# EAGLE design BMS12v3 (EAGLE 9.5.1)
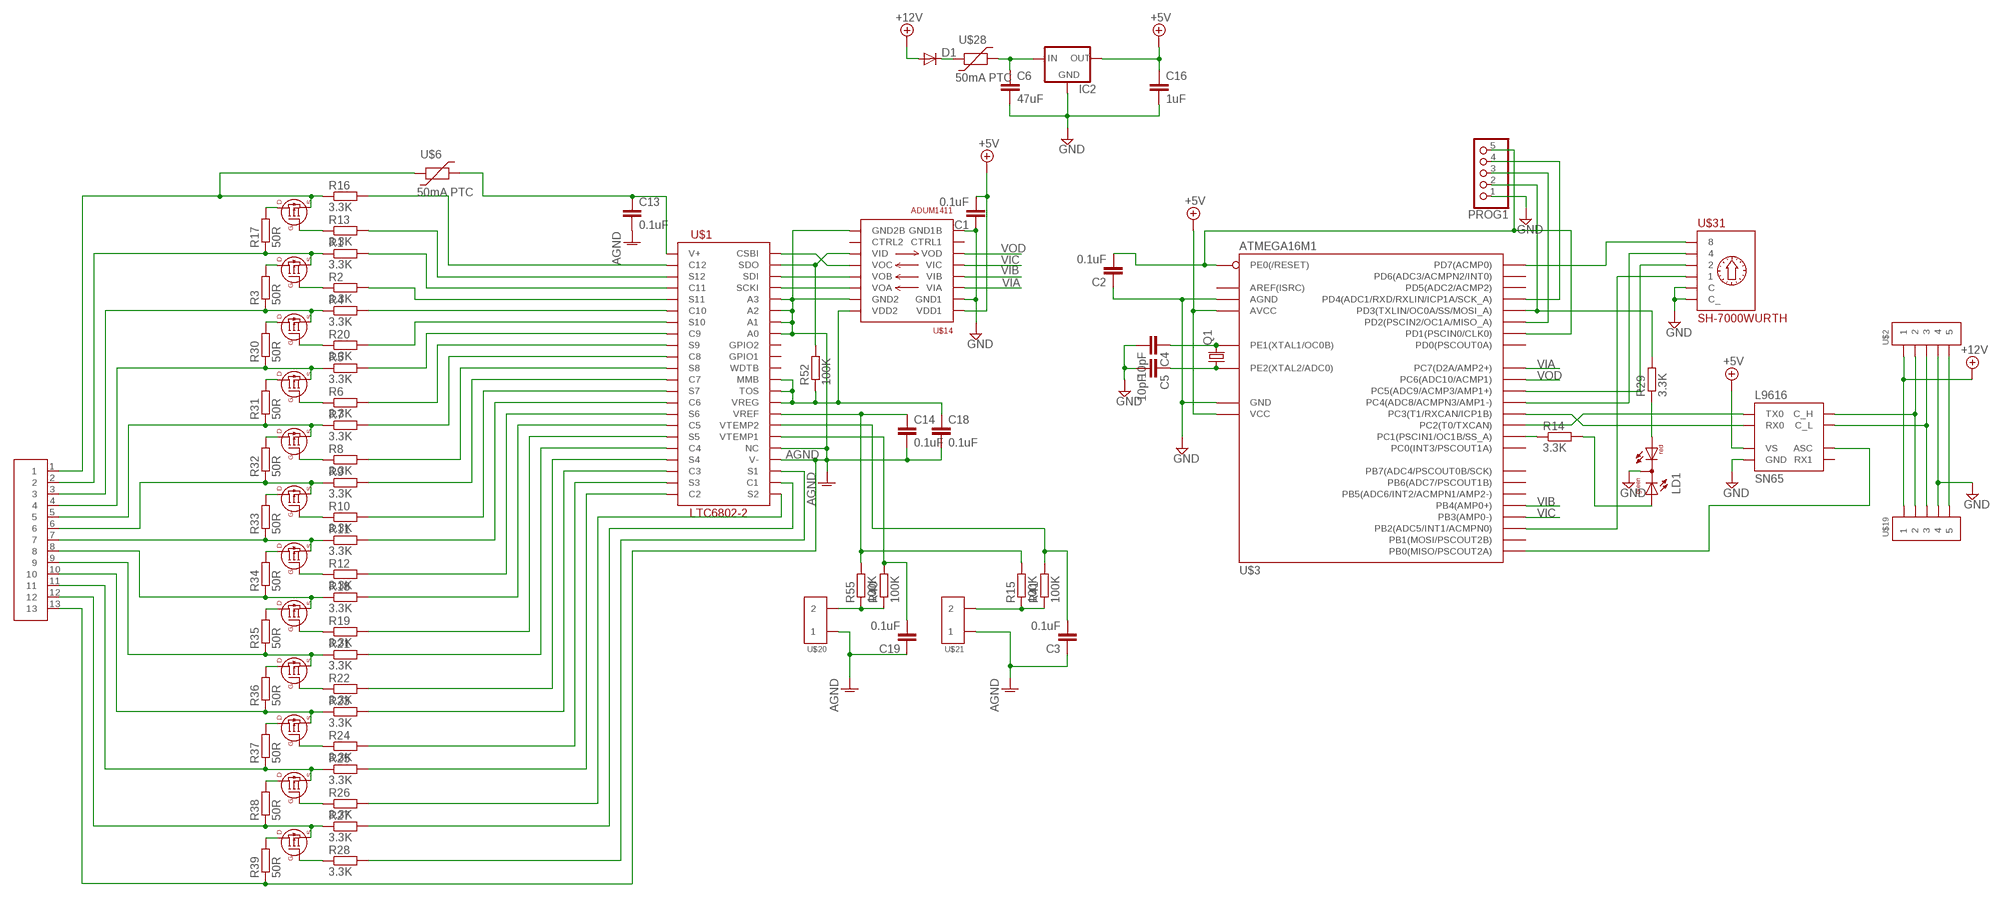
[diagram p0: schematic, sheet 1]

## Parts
C1  0.1uF  C-EUC0805  [C0805]
C2  0.1uF  C-EUC0805  [C0805]
C3  0.1uF  C-EUC0805  [C0805]
C4  10pF  C-EUC0805  [C0805]
C5  10pF  C-EUC0805  [C0805]
C6  47uF  C-EUC1206  [C1206]
C13  0.1uF  C-EUC0805  [C0805]
C14  0.1uF  C-EUC0805  [C0805]
C16  1uF  C-EUC0805  [C0805]
C18  0.1uF  C-EUC0805  [C0805]
C19  0.1uF  C-EUC0805  [C0805]
D1  DIODE-SOD123  [SOD123]
IC2  78LXXSOT89  [SOT89R]
LD1  DUOLED-RG-C  [DUOLED-C-5MM]
PROG1  PINHD-1X5  [1X05]
Q1  CRYSTALCTS406  [CTS406]
R1  3.3K  R-EU_R0805  [R0805]
R2  3.3K  R-EU_R0805  [R0805]
R3  50R  R-EU_R2512  [R2512]
R4  3.3K  R-EU_R0805  [R0805]
R5  3.3K  R-EU_R0805  [R0805]
R6  3.3K  R-EU_R0805  [R0805]
R7  3.3K  R-EU_R0805  [R0805]
R8  3.3K  R-EU_R0805  [R0805]
R9  3.3K  R-EU_R0805  [R0805]
R10  3.3K  R-EU_R0805  [R0805]
R11  3.3K  R-EU_R0805  [R0805]
R12  3.3K  R-EU_R0805  [R0805]
R13  3.3K  R-EU_R0805  [R0805]
R14  3.3K  R-EU_R0805  [R0805]
R15  100K  R-EU_R0805  [R0805]
R16  3.3K  R-EU_R0805  [R0805]
R17  50R  R-EU_R2512  [R2512]
R18  3.3K  R-EU_R0805  [R0805]
R19  3.3K  R-EU_R0805  [R0805]
R20  3.3K  R-EU_R0805  [R0805]
R21  3.3K  R-EU_R0805  [R0805]
R22  3.3K  R-EU_R0805  [R0805]
R23  3.3K  R-EU_R0805  [R0805]
R24  3.3K  R-EU_R0805  [R0805]
R25  3.3K  R-EU_R0805  [R0805]
R26  3.3K  R-EU_R0805  [R0805]
R27  3.3K  R-EU_R0805  [R0805]
R28  3.3K  R-EU_R0805  [R0805]
R29  3.3K  R-EU_R0805  [R0805]
R30  50R  R-EU_R2512  [R2512]
R31  50R  R-EU_R2512  [R2512]
R32  50R  R-EU_R2512  [R2512]
R33  50R  R-EU_R2512  [R2512]
R34  50R  R-EU_R2512  [R2512]
R35  50R  R-EU_R2512  [R2512]
R36  50R  R-EU_R2512  [R2512]
R37  50R  R-EU_R2512  [R2512]
R38  50R  R-EU_R2512  [R2512]
R39  50R  R-EU_R2512  [R2512]
R40  100K  R-EU_R0805  [R0805]
R41  100K  R-EU_R0805  [R0805]
R52  100K  R-EU_R0805  [R0805]
R55  100K  R-EU_R0805  [R0805]
SN65  L9616  [SOIC8]
U$1  LTC6802-2  [SSOP-44]
U$2  MOLEX-39502-1005  [MOLEX-39502-1005]
U$3  ATMEGA16M1  [TQFP32]
U$4  SI2351DS  [SOT23]
U$5  SI2351DS  [SOT23]
U$6  50mA PTC  1206_POLYSWITCH  [1206]
U$7  SI2351DS  [SOT23]
U$8  SI2351DS  [SOT23]
U$9  SI2351DS  [SOT23]
U$10  SI2351DS  [SOT23]
U$11  SI2351DS  [SOT23]
U$12  SI2351DS  [SOT23]
U$13  SI2351DS  [SOT23]
U$14  ADUM1411  [SOIC16W]
U$15  SI2351DS  [SOT23]
U$16  SI2351DS  [SOT23]
U$17  SI2351DS  [SOT23]
U$18  MOLEX_TERM_BLOCK_13  [MOLEX_TERM_BLOCK_13]
U$19  MOLEX-39502-1005  [MOLEX-39502-1005]
U$20  MOLEX-39502-1002  [MOLEX-39502-1002]
U$21  MOLEX-39502-1002  [MOLEX-39502-1002]
U$28  50mA PTC  1206_POLYSWITCH  [1206]
U$31  SH-7000WURTH  [WS-ROTV]

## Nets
+5V: C1.2 C16.1 IC2.2(OUT) SN65.P$3(VS) U$3.4(VCC) U$3.19(AVCC) U$14.1(VDD1)
+12V: D1.A U$2.1 U$19.1
AGND: C3.1 C13.2 C14.2 C18.2 C19.1 R39.1 U$1.26(V-) U$1.27(NC) U$1.37(A0) U$1.38(A1) U$1.39(A2) U$1.40(A3) U$14.9(GND2B) U$14.15(GND2) U$18.13 U$20.1 U$21.1
GND: C1.1 C2.1 C4.2 C5.2 C6.2 C16.2 IC2.4(GND) LD1.C PROG1.1 SN65.P$2(GND) U$2.4 U$3.5(GND) U$3.20(AGND) U$14.2(GND1) U$14.8(GND1B) U$19.4 U$31.C U$31.C2(C_)
N$1: D1.C U$28.P$1
N$2: R16.2 U$1.2(C12)
N$3: R13.2 U$1.3(S12)
N$4: R3.2 U$5.P$3(D)
N$5: R1.2 U$1.4(C11)
N$6: R1.1 R17.1 U$5.P$2(S) U$18.2
N$7: U$1.42(SDI) U$14.13(VOB)
N$8: R3.1 R4.1 U$7.P$2(S) U$18.3
N$9: R4.2 U$1.6(C10)
N$10: R26.2 U$1.23(S2)
N$11: U$1.41(SCKI) U$14.14(VOA)
N$12: R27.2 U$1.24(C1)
N$13: R28.2 U$1.25(S1)
N$14: R2.2 U$1.5(S11)
N$15: R52.2 U$1.43(SDO) U$14.11(VID)
N$16: U$1.44(CSBI) U$14.12(VOC)
N$17: R2.1 U$5.P$1(G)
N$18: R30.2 U$7.P$3(D)
N$19: C2.2 PROG1.5 U$3.31(PE0(/RESET)) U$3.32(PD1(PSCIN0/CLK0))
N$20: C6.1 IC2.1(IN) U$28.P$2
N$21: R5.2 U$1.8(C9)
N$22: R7.2 U$1.10(C8)
N$23: R9.2 U$1.12(C7)
N$24: R11.2 U$1.14(C6)
N$25: C18.1 R52.1 U$1.31(VREG) U$1.32(TOS) U$1.33(MMB) U$14.16(VDD2)
N$26: R18.2 U$1.16(C5)
N$27: R21.2 U$1.18(C4)
N$28: R23.2 U$1.20(C3)
N$29: R25.2 U$1.22(C2)
N$30: SN65.P$8(ASC) U$3.8(PB0(MISO/PSCOUT2A))
N$31: R5.1 R30.1 U$8.P$2(S) U$18.4
N$32: PROG1.2 R29.2 U$3.2(PD3(TXLIN/OC0A/SS/MOSI_A))
N$33: PROG1.3 U$3.1(PD2(PSCIN2/OC1A/MISO_A))
N$34: PROG1.4 U$3.12(PD4(ADC1/RXD/RXLIN/ICP1A/SCK_A))
N$36: SN65.P$4(RX0) U$3.7(PC3(T1/RXCAN/ICP1B))
N$37: SN65.P$1(TX0) U$3.6(PC2(T0/TXCAN))
N$38: SN65.P$7(C_H) U$2.2 U$19.2
N$39: SN65.P$6(C_L) U$2.3 U$19.3
N$40: LD1.AX(AG) R14.2
N$41: R14.1 U$3.3(PC1(PSCIN1/OC1B/SS_A))
N$42: U$3.15(PD7(ACMP0)) U$31.8
N$43: U$3.16(PB2(ADC5/INT1/ACMPN0)) U$31.1
N$44: U$3.17(PC4(ADC8/ACMPN3/AMP1-)) U$31.4
N$45: U$3.18(PC5(ADC9/ACMP3/AMP1+)) U$31.2
N$46: C3.2 R41.2 U$1.29(VTEMP2)
N$47: U$2.5 U$19.5
N$48: C4.1 Q1.3 U$3.10(PE1(XTAL1/OC0B))
N$49: C5.1 Q1.1 U$3.11(PE2(XTAL2/ADC0))
N$50: R17.2 U$4.P$3(D)
N$51: R16.1 U$4.P$2(S) U$6.P$1 U$18.1
N$52: R13.1 U$4.P$1(G)
N$53: R7.1 R31.1 U$9.P$2(S) U$18.5
N$54: R31.2 U$8.P$3(D)
N$55: R6.1 U$8.P$1(G)
N$56: R20.1 U$7.P$1(G)
N$57: R8.1 U$9.P$1(G)
N$58: R10.1 U$10.P$1(G)
N$59: R12.1 U$11.P$1(G)
N$60: R28.1 U$17.P$1(G)
N$61: R19.1 U$12.P$1(G)
N$62: R22.1 U$13.P$1(G)
N$63: R24.1 U$15.P$1(G)
N$64: R26.1 U$16.P$1(G)
N$65: R27.1 R38.1 U$17.P$2(S) U$18.12
N$66: C14.1 R15.2 R55.2 U$1.30(VREF)
N$67: C19.2 R40.2 U$1.28(VTEMP1)
N$68: LD1.AR R29.1
N$69: R25.1 R37.1 U$16.P$2(S) U$18.11
N$70: R23.1 R36.1 U$15.P$2(S) U$18.10
N$71: R38.2 U$16.P$3(D)
N$72: R39.2 U$17.P$3(D)
N$73: R37.2 U$15.P$3(D)
N$74: R21.1 R35.1 U$13.P$2(S) U$18.9
N$75: R36.2 U$13.P$3(D)
N$76: R18.1 R34.1 U$12.P$2(S) U$18.8
N$77: R35.2 U$12.P$3(D)
N$78: R11.1 R33.1 U$11.P$2(S) U$18.7
N$79: R9.1 R32.1 U$10.P$2(S) U$18.6
N$80: R33.2 U$10.P$3(D)
N$81: R34.2 U$11.P$3(D)
N$82: R32.2 U$9.P$3(D)
N$83: R24.2 U$1.21(S3)
N$84: R22.2 U$1.19(S4)
N$85: R40.1 R55.1 U$20.2
N$86: R15.1 R41.1 U$21.2
N$87: R20.2 U$1.7(S10)
N$88: R6.2 U$1.9(S9)
N$89: R8.2 U$1.11(S8)
N$90: R10.2 U$1.13(S7)
N$91: R12.2 U$1.15(S6)
N$93: R19.2 U$1.17(S5)
V+: C13.1 U$1.1(V+) U$6.P$2
VIA: U$3.25(PC7(D2A/AMP2+)) U$14.3(VIA)
VIB: U$3.24(PB4(AMP0+)) U$14.4(VIB)
VIC: U$3.23(PB3(AMP0-)) U$14.5(VIC)
VOD: U$3.22(PC6(ADC10/ACMP1)) U$14.6(VOD)
Unconnected: SN65.P$5(RX1) U$1.34(WDTB) U$1.35(GPIO1) U$1.36(GPIO2) U$3.9(PB1(MOSI/PSCOUT2B)) U$3.13(PD5(ADC2/ACMP2)) U$3.14(PD6(ADC3/ACMPN2/INT0)) U$3.21(AREF(ISRC)) U$3.26(PB5(ADC6/INT2/ACMPN1/AMP2-)) U$3.27(PB6(ADC7/PSCOUT1B)) U$3.28(PB7(ADC4/PSCOUT0B/SCK)) U$3.29(PD0(PSCOUT0A)) U$3.30(PC0(INT3/PSCOUT1A)) U$14.7(CTRL1) U$14.10(CTRL2)

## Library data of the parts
C1-C6 C13 C14 C16 C18 C19 = resistor:C-EU: CAPACITOR, European symbol
D1 = diode:DIODE-: DIODE
IC2 = v-reg:78LXX: VOLTAGE REGULATOR
LD1 = led:DUOLED-RG-C: DUO LED 2 colors (red/green), 5 mm, round, common Cathode www.ligitek.com or other producers.
PROG1 = pinhead:PINHD-1X5: PIN HEADER
Q1 = crystal:CRYSTAL: CRYSTAL
R1-R41 R52 R55 = resistor:R-EU_: RESISTOR, European symbol
SN65 = Ians parts:L9616
U$1 = Ians parts:LTC6802-2
U$2 U$19 = Ians parts:MOLEX-39502-1005
U$3 = Ians parts:ATMEGA16M1
U$4 U$5 U$7-U$13 U$15-U$17 = Ians parts:SI2351DS
U$6 U$28 = Ians parts:1206_POLYSWITCH
U$14 = Ians parts:ADUM1411
U$18 = Ians parts:MOLEX_TERM_BLOCK_13
U$20 U$21 = Ians parts:MOLEX-39502-1002
U$31 = Ians parts:SH-7000

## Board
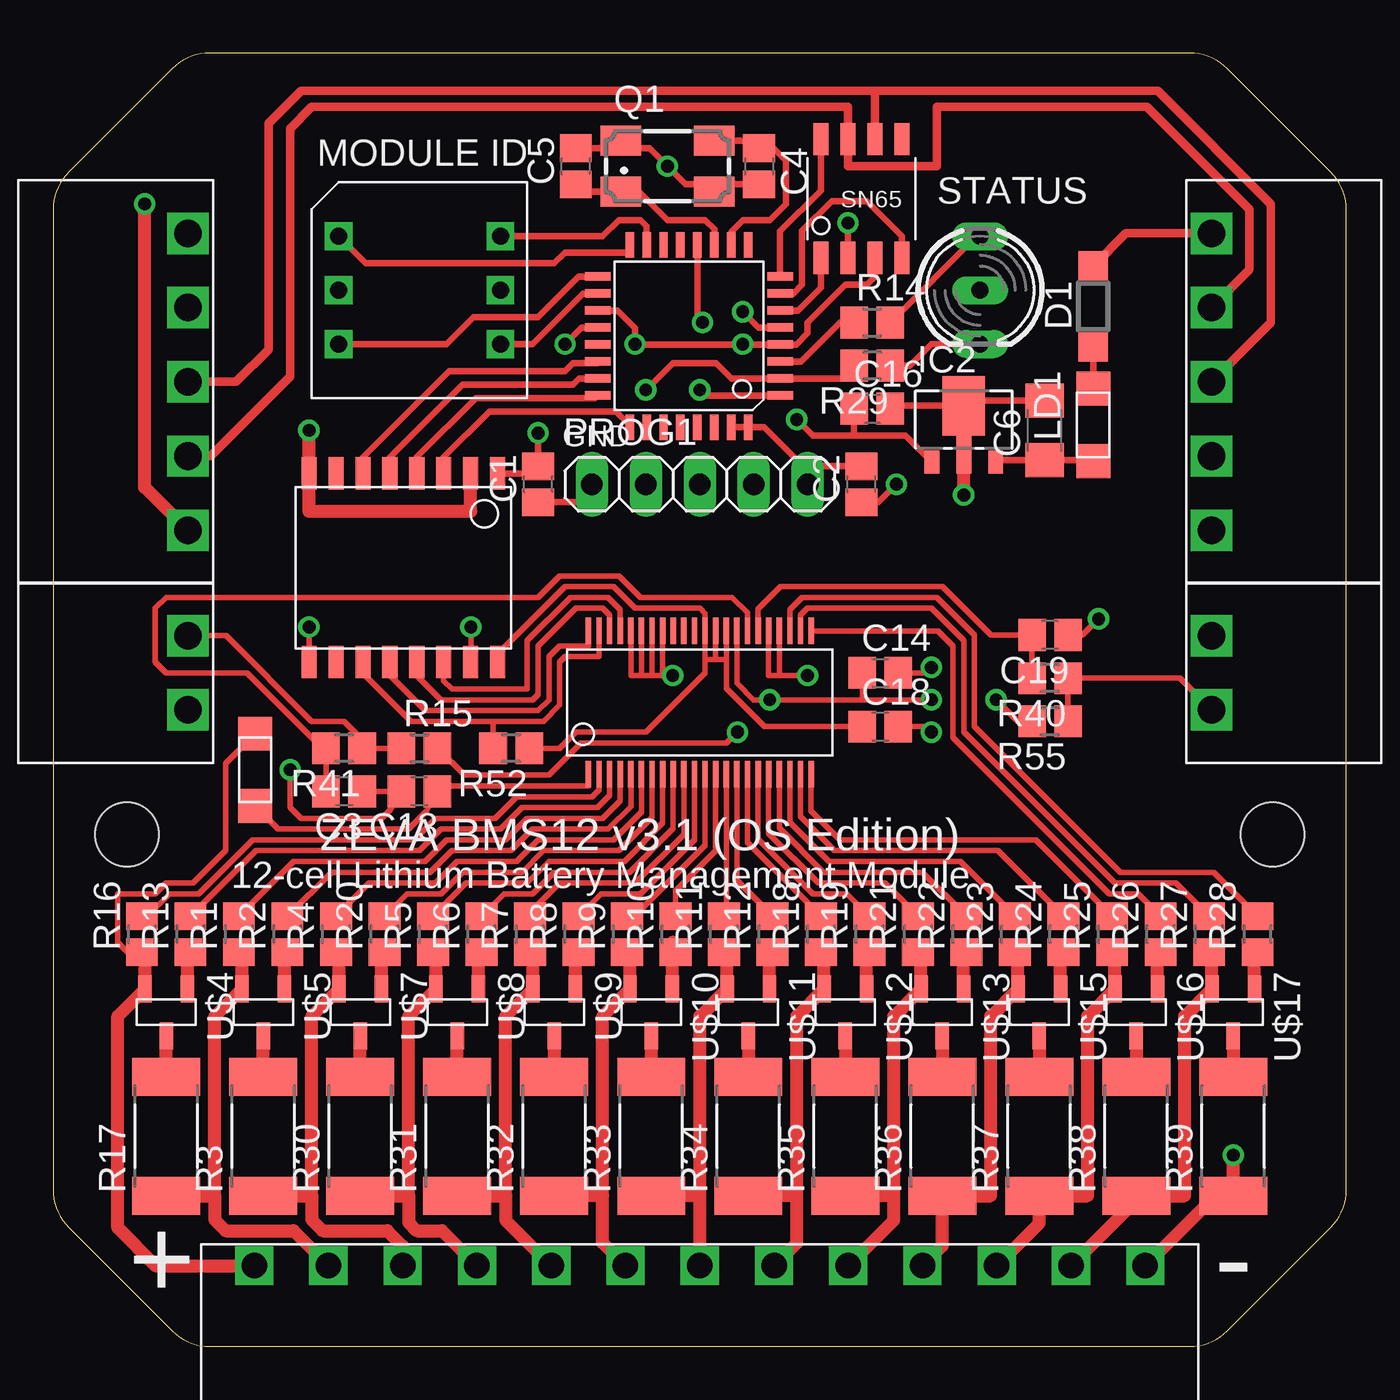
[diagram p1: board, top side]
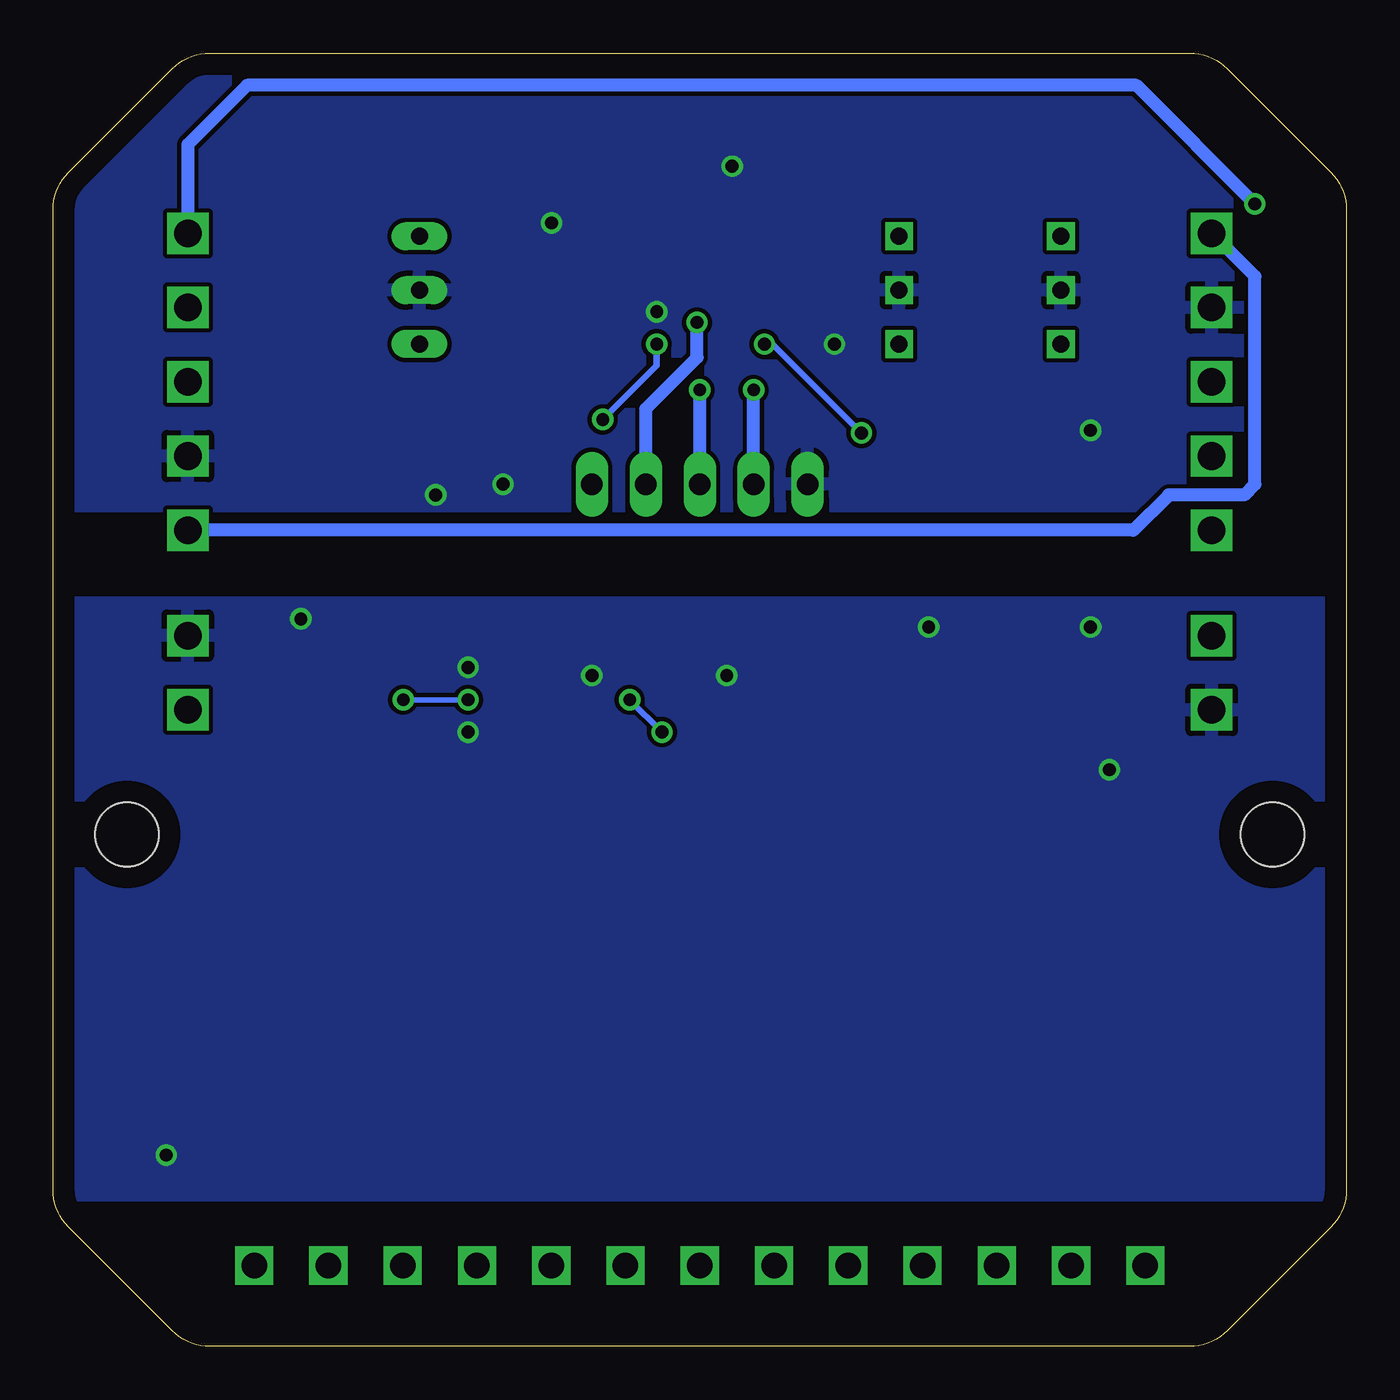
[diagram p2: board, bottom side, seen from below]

Size 60.96 x 60.96 mm. Coordinates in mm from the lower left corner, seen from the top.
Outline: 5.61,0.74 arc45 7.4,0 53.56,0 arc45 55.35,0.74 60.22,5.61 arc45 60.96,7.4 60.96,53.56 arc45 60.22,55.35 55.35,60.22 arc45 53.56,60.96 7.4,60.96 arc45 5.61,60.22 0.74,55.35 arc45 0,53.56 0,7.4 arc45 0.74,5.61 5.61,0.74
Copper layers (1*16): Top 0.035mm / dielectric 1.5mm / Bottom 0.035mm
Design rules "default *": minimum track width 10mil, minimum drill 10mil, track to track 8mil, track to pad 8mil, pad to pad 8mil, via to via 8mil, smd to smd 8mil, copper to edge 40mil, drill to drill 8mil, minimum pad ring 10mil, minimum via ring 8mil, stop-mask expansion 4mil, vias tented up to drill 0mil, thermal gap 10mil
Holes 3 mm at 3.48,24.13 57.48,24.13

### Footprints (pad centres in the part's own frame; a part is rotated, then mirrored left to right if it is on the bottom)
C0805 = smd 1.3 x 1.5: 1 -0.85,0; 2 0.85,0
C1206 = smd 1.6 x 1.8: 1 -1.4,0; 2 1.4,0
SOD123 = smd 1.4 x 1.4: A 1.9,0; C -1.9,0
SOT89R = smd 0.7 x 1.1: 1 1.5,-1.75; 2 -1.5,-1.75 | smd 0.7 x 1.8: 3 0,-1.4 | smd 2 x 2.8: 4 0,0.9
DUOLED-C-5MM = drill 0.813 long: AR 2.54,0; AX -2.54,0; C 0,0
1X05 = drill 1.016 long: 1 -5.08,0; 2 -2.54,0; 3 0,0; 4 2.54,0; 5 5.08,0
CTS406 = smd 1.9 x 1.4: 1 -2.2,-1.2; 2 2.2,-1.2; 3 2.2,1.2; 4 -2.2,1.2
R0805 = smd 1.3 x 1.5: 1 -0.85,0; 2 0.85,0
R2512 = smd 1.8 x 3.2: 1 -2.8,0; 2 2.8,0
SOIC8 = smd 1.524 x 0.711: P$1 -2.794,1.905; P$2 -2.794,0.635; P$3 -2.794,-0.635; P$4 -2.794,-1.905; P$5 2.794,-1.905; P$6 2.794,-0.635; P$7 2.794,0.635; P$8 2.794,1.905
SSOP-44 = smd 1.25 x 0.25: 1 -3.375,5.25; 2 -3.375,4.75; 3 -3.375,4.25; 4 -3.375,3.75; 5 -3.375,3.25; 6 -3.375,2.75; 7 -3.375,2.25; 8 -3.375,1.75; 9 -3.375,1.25; 10 -3.375,0.75; 11 -3.375,0.25; 12 -3.375,-0.25; 13 -3.375,-0.75; 14 -3.375,-1.25; 15 -3.375,-1.75; 16 -3.375,-2.25; 17 -3.375,-2.75; 18 -3.375,-3.25; 19 -3.375,-3.75; 20 -3.375,-4.25; 21 -3.375,-4.75; 22 -3.375,-5.25; 23 3.375,-5.25; 24 3.375,-4.75; 25 3.375,-4.25; 26 3.375,-3.75; 27 3.375,-3.25; 28 3.375,-2.75; 29 3.375,-2.25; 30 3.375,-1.75; 31 3.375,-1.25; 32 3.375,-0.75; 33 3.375,-0.25; 34 3.375,0.25; 35 3.375,0.75; 36 3.375,1.25; 37 3.375,1.75; 38 3.375,2.25; 39 3.375,2.75; 40 3.375,3.25; 41 3.375,3.75; 42 3.375,4.25; 43 3.375,4.75; 44 3.375,5.25
MOLEX-39502-1005 = drill 1.3 square: 1 -7,0; 2 -3.5,0; 3 0,0; 4 3.5,0; 5 7,0
TQFP32 = smd 1.2 x 0.4: 1 -4.3,2.8; 2 -4.3,2; 3 -4.3,1.2; 4 -4.3,0.4; 5 -4.3,-0.4; 6 -4.3,-1.2; 7 -4.3,-2; 8 -4.3,-2.8; 17 4.3,-2.8; 18 4.3,-2; 19 4.3,-1.2; 20 4.3,-0.4; 21 4.3,0.4; 22 4.3,1.2; 23 4.3,2; 24 4.3,2.8 | smd 0.4 x 1.2: 9 -2.8,-4.3; 10 -2,-4.3; 11 -1.2,-4.3; 12 -0.4,-4.3; 13 0.4,-4.3; 14 1.2,-4.3; 15 2,-4.3; 16 2.8,-4.3; 25 2.8,4.3; 26 2,4.3; 27 1.2,4.3; 28 0.4,4.3; 29 -0.4,4.3; 30 -1.2,4.3; 31 -2,4.3; 32 -2.8,4.3
SOT23 = smd 1.27 x 0.635: P$1 -1.1,1; P$2 -1.1,-1; P$3 1.1,0
1206 = smd 1.6 x 1.6: P$1 -1.7,0; P$2 1.7,0
SOIC16W = smd 1.524 x 0.711: 1 -4.445,4.445; 2 -4.445,3.175; 3 -4.445,1.905; 4 -4.445,0.635; 5 -4.445,-0.635; 6 -4.445,-1.905; 7 -4.445,-3.175; 8 -4.445,-4.445; 9 4.445,-4.445; 10 4.445,-3.175; 11 4.445,-1.905; 12 4.445,-0.635; 13 4.445,0.635; 14 4.445,1.905; 15 4.445,3.175; 16 4.445,4.445
MOLEX_TERM_BLOCK_13 = drill 1.2 square: 1 -21,0; 2 -17.5,0; 3 -14,0; 4 -10.5,0; 5 -7,0; 6 -3.5,0; 7 0,0; 8 3.5,0; 9 7,0; 10 10.5,0; 11 14,0; 12 17.5,0; 13 21,0
MOLEX-39502-1002 = drill 1.3 square: 1 -1.75,0; 2 1.75,0
WS-ROTV = drill 0.8 square: 1 -3.81,2.54; 2 3.81,-2.54; 4 -3.81,-2.54; 8 3.81,2.54; C -3.81,0; C2 3.81,0

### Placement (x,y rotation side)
C1  22.86,40.64 90 top
C2  38.1,40.64 90 top
C3  13.72,26.16 180 top
C4  33.27,55.63 270 top
C5  24.64,55.63 90 top
C6  46.74,43.18 90 top
C13  17.27,26.16 180 top
C14  38.99,31.75 0 top
C16  38.61,44.2 0 top
C18  38.99,29.21 0 top
C19  46.99,33.53 180 top
D1  49.02,49.02 90 top
IC2  42.93,43.43 0 top
LD1  43.69,49.78 270 top
PROG1  30.48,40.64 0 top
Q1  28.96,55.63 0 top
R1  8.76,19.43 90 top
R2  11.05,19.43 90 top
R3  9.91,9.91 90 top
R4  13.34,19.43 90 top
R5  17.91,19.43 90 top
R6  20.19,19.43 90 top
R7  22.48,19.43 90 top
R8  24.77,19.43 90 top
R9  27.05,19.43 90 top
R10  29.34,19.43 90 top
R11  31.62,19.43 90 top
R12  33.91,19.43 90 top
R13  6.48,19.43 90 top
R14  38.61,48.26 0 top
R15  17.27,28.19 0 top
R16  4.19,19.43 90 top
R17  5.33,9.91 90 top
R18  36.2,19.43 90 top
R19  38.48,19.43 90 top
R20  15.62,19.43 90 top
R21  40.77,19.43 90 top
R22  43.05,19.43 90 top
R23  45.34,19.43 90 top
R24  47.62,19.43 90 top
R25  49.91,19.43 90 top
R26  52.2,19.43 90 top
R27  54.48,19.43 90 top
R28  56.77,19.43 90 top
R29  38.61,46.23 180 top
R30  14.48,9.91 90 top
R31  19.05,9.91 90 top
R32  23.62,9.91 90 top
R33  28.19,9.91 90 top
R34  32.77,9.91 90 top
R35  37.34,9.91 90 top
R36  41.91,9.91 90 top
R37  46.48,9.91 90 top
R38  51.05,9.91 90 top
R39  55.63,9.91 90 top
R40  46.99,31.5 180 top
R41  13.72,28.19 180 top
R52  21.59,28.19 180 top
R55  46.99,29.46 180 top
SN65  38.1,54.1 90 top
U$1  30.48,30.35 90 top
U$2  6.35,45.47 90 top
U$3  29.97,47.62 180 top
U$4  5.33,15.75 270 top
U$5  9.91,15.75 270 top
U$6  9.53,27.18 270 top
U$7  14.48,15.75 270 top
U$8  19.05,15.75 270 top
U$9  23.62,15.75 270 top
U$10  28.19,15.75 270 top
U$11  32.77,15.75 270 top
U$12  37.34,15.75 270 top
U$13  41.91,15.75 270 top
U$14  16.51,36.7 270 top
U$15  46.48,15.75 270 top
U$16  51.05,15.75 270 top
U$17  55.63,15.75 270 top
U$18  30.48,3.81 0 top
U$19  54.61,45.47 270 top
U$20  54.61,31.75 270 top
U$21  6.35,31.75 90 top
U$28  49.02,43.43 270 top
U$31  17.27,49.78 0 top

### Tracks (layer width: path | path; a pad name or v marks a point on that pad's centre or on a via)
+5V  (via drill 0.6)
  Top 0.305: v22.86,43.05 C1.2 22.86,41.15 U$14.1 | SN65.P$3 38.73,50.42 38.35,50.04 37.34,50.04 35.56,48.26 35.56,47.75 35.03,47.23 U$3.4 32.51,47.23 | U$3.19 26.61,48.83 27.43,48.01 v27.43,47.24 27.45,47.23 32.51,47.23 | 32.51,47.23 v32.51,47.24 | v35.05,43.69 35.81,42.93 36.58,42.93 37.76,42.93 | 37.76,42.93 40.18,42.93 IC2.2 | 37.76,42.93 C16.1
  Bottom 0.305: v27.43,47.24 27.05,47.24 v22.86,43.05 | v32.51,47.24 32.51,46.23 v35.05,43.69
+12V  (via drill 0.6)
  Top 0.406: U$19.1 50.57,52.47 D1.A
  Top 0.61: U$2.1 4.32,40.5 v4.32,53.85
  Bottom 0.61: v4.32,53.85 9.91,59.44 51.82,59.44 54.61,56.64 U$19.1
AGND  (via drill 0.6)
  Top 0.254: 34.23,31.62 U$1.26 | 34.23,31.62 v35.56,31.62 | U$1.27 33.73,31.62 34.23,31.62 | U$1.37 28.73,31.62 v29.21,31.62 | U$1.38 28.23,31.62 v29.21,31.62 | U$1.39 27.73,31.62 v29.21,31.62 | U$1.40 27.23,31.62 v29.21,31.62 | U$14.15 v19.69,33.91 | U$14.9 v12.06,33.91 | C14.2 41.15,31.75 v41.4,32 | C18.2 41.15,29.21 v41.4,28.96 | C19.1 48.51,33.53 v49.28,34.29 | C3.1 C13.2 15.91,25.31 15.49,24.89 11.68,24.89 11.18,25.4 v11.18,27.18
  Top 0.61: U$18.13 54.78,7.11 R39.1 v55.63,9.02
  Bottom 0.61: v12.06,33.91 11.81,33.91
  pour Bottom: -1.52,7.11 61.98,7.11 62.23,35.05 -1.27,35.05
GND  (via drill 0.6)
  Top 0.305: U$3.5 33.26,48.02 v32.51,48.77 | SN65.P$2 v37.47,52.96 | v39.75,40.64 38.9,39.79 C2.1 | C1.1 25.4,39.79 PROG1.1 | C5.2 28.11,56.48 v28.96,55.63 29.81,54.78 C4.2 | C6.2 43.17,44.58 IC2.4 39.46,44.33 C16.2 | U$3.20 24.91,48.02 v24.13,47.24
  Top 0.61: U$14.2 19.68,39.37 12.06,39.37 U$14.8 v12.06,43.18 | v42.93,40.13 IC2.4
  pour Bottom: -1.27,39.62 -1.27,62.23 62.23,62.23 62.23,39.62
N$1
  Top 0.305: U$28.P$1 D1.C
N$2
  Top 0.254: U$1.2 25.73,26.24 25.4,25.91 21.84,25.91 20.83,24.89 18.03,24.89 17.02,23.88 9.4,23.88 6.86,21.34 5.5,21.34 4.45,20.28 R16.2
N$3
  Top 0.254: U$1.3 26.23,25.98 25.65,25.4 22.1,25.4 21.08,24.38 18.29,24.38 17.27,23.37 9.56,23.37 R13.2
N$4
  Top 0.61: R3.2 U$5.P$3
N$5
  Top 0.254: U$1.4 26.73,25.71 25.91,24.89 22.35,24.89 21.34,23.88 18.54,23.88 17.53,22.86 11.34,22.86 R1.2
N$6
  Top 0.61: U$18.2 11.33,5.46 8.13,5.46 7.62,5.97 7.62,7.11 | 7.62,7.11 7.62,15.56 U$5.P$2 8.91,18.44 R1.1 | R17.1 7.62,7.11
N$7
  Top 0.254: U$1.42 26.23,34.48 25.91,34.8 24.64,34.8 22.86,33.02 22.86,30.73 22.61,30.48 18.29,30.48 17.14,31.62 U$14.13
N$8
  Top 0.61: 12.19,7.11 12.19,15.56 U$7.P$2 13.48,18.44 R4.1 | U$18.3 16.48,4.73 15.75,5.46 12.7,5.46 12.19,5.97 12.19,7.11 | R3.1 12.19,7.11
N$9
  Top 0.254: U$1.6 27.73,25.19 26.42,23.88 22.86,23.88 21.84,22.86 19.05,22.86 18.03,21.84 14.9,21.84 R4.2
N$10
  Top 0.254: U$1.23 41.71,33.73 42.42,33.02 42.42,28.7 49.78,21.34 51.14,21.34 R26.2
N$11
  Top 0.254: U$1.41 26.73,34.74 26.16,35.31 24.38,35.31 22.35,33.27 22.35,30.99 18.8,30.99 18.41,31.37 U$14.14
N$12
  Top 0.254: U$1.24 35.23,34.47 35.56,34.8 41.4,34.8 42.93,33.27 42.93,28.96 50.04,21.84 52.92,21.84 R27.2
N$13
  Top 0.254: U$1.25 34.73,34.73 35.31,35.31 41.66,35.31 43.43,33.53 43.43,29.21 50.29,22.35 54.7,22.35 R28.2
N$14
  Top 0.254: U$1.5 27.23,25.45 26.16,24.38 22.61,24.38 21.59,23.37 18.8,23.37 17.78,22.35 13.12,22.35 R2.2
N$15
  Top 0.254: U$1.43 25.73,32.51 24.13,32.51 23.88,32.26 23.88,30.23 23.11,29.46 20.74,29.46 | U$14.11 14.61,31.73 16.87,29.46 20.74,29.46 | 20.74,29.46 R52.2
N$16
  Top 0.254: U$1.44 25.23,33.02 23.88,33.02 23.37,32.51 23.37,30.48 22.86,29.97 17.53,29.97 15.88,31.62 U$14.12
N$17
  Top 0.61: R2.1 10.91,18.44 U$5.P$1
N$18
  Top 0.61: R30.2 U$7.P$3
N$19
  Top 0.305: U$3.31 U$3.32 33.51,43.33 35.56,41.27 PROG1.5 35.56,41.49 C2.2
N$20
  Top 0.305: U$28.P$2 48.98,41.78 C6.1 44.52,41.78 IC2.1
N$21
  Top 0.254: U$1.8 28.73,24.67 26.92,22.86 23.37,22.86 22.35,21.84 19.47,21.84 R5.2
N$22
  Top 0.254: U$1.10 29.73,24.14 27.43,21.84 23.88,21.84 22.48,20.45 R7.2
N$23
  Top 0.254: U$1.12 30.73,23.62 27.69,20.57 27.34,20.57 R9.2
N$24
  Top 0.254: U$1.14 31.73,20.39 R11.2
N$25
  Top 0.254: 31.73,32.38 U$1.31 | 31.23,32.38 U$1.32 | 31.23,32.38 31.73,32.38 | 30.73,32.38 U$1.33 30.73,34.55 30.48,34.8 27.43,34.8 26.42,35.81 24.13,35.81 20.95,32.64 U$14.16 | 30.73,32.38 31.23,32.38 | 30.73,32.38 30.73,31.75 27.94,28.96 24.64,28.96 23.88,28.19 R52.1 | C18.1 33.53,29.21 31.73,31.01 31.73,32.38
N$26
  Top 0.254: U$1.16 32.73,23.75 R18.2
N$27
  Top 0.254: U$1.18 33.73,24.18 36.07,21.84 39.2,21.84 R21.2
N$28
  Top 0.254: U$1.20 34.73,24.71 36.58,22.86 42.76,22.86 R23.2
N$29
  Top 0.254: U$1.22 35.73,25.23 37.08,23.88 46.32,23.88 R25.2
N$30
  Top 0.305: SN65.P$8 36.2,54.48 34.27,52.56 U$3.8
N$31
  Top 0.61: 16.76,7.11 16.76,15.56 U$8.P$2 18.05,18.44 R5.1 | U$18.4 18.33,5.46 17.14,5.46 16.76,5.84 16.76,7.11 | R30.1 16.76,7.11
N$32  (via drill 0.6)
  Top 0.305: v27.94,45.09 29.21,46.35 31.24,46.35 31.97,45.62 U$3.2 37.16,45.62 R29.2
  Bottom 0.61: PROG1.2 v27.94,45.09
N$33  (via drill 0.6)
  Top 0.305: U$3.1 30.73,44.83 v30.48,45.09
  Bottom 0.61: PROG1.3 v30.48,45.09
N$34  (via drill 0.6)
  Top 0.305: U$3.12 30.37,48.49 v30.61,48.26
  Bottom 0.61: PROG1.4 33.02,44.2 30.61,46.61 v30.61,48.26
N$36
  Top 0.305: SN65.P$4 40.01,52.32 38.35,53.98 36.7,53.98 35.31,52.58 35.31,50.04 34.89,49.62 U$3.7
N$37
  Top 0.305: U$3.6 35.11,48.83 36.2,49.91 SN65.P$1
N$38
  Top 0.406: U$2.2 7.42,41.97 11.18,45.72 11.18,57.4 12.19,58.42 37.47,58.42 SN65.P$7 37.47,55.63 41.66,55.63 41.66,58.42 51.56,58.42 56.39,53.59 56.39,50.74 U$19.2
N$39
  Top 0.406: 38.73,59.18 SN65.P$6 | 38.73,59.18 52.07,59.18 57.4,53.85 57.4,48.26 U$19.3 | U$2.3 8.64,45.47 10.16,46.99 10.16,57.66 11.68,59.18 38.73,59.18
N$40
  Top 0.305: LD1.AX 43.52,52.32 R14.2
N$41
  Top 0.305: R14.1 37.08,48.26 35.25,46.42 U$3.3
N$42
  Top 0.305: U$3.15 27.97,52.8 27.69,53.09 26.67,53.09 25.91,52.32 U$31.8
N$43
  Top 0.305: U$31.1 14.73,51.05 23.62,51.05 24.13,51.56 27.17,51.56 U$3.16
N$44
  Top 0.305: U$3.17 24.77,50.42 22.86,48.51 19.81,48.51 18.54,47.24 U$31.4
N$45
  Top 0.305: U$3.18 24.99,49.62 22.61,47.24 U$31.2
N$46
  Top 0.254: U$1.29 32.73,34.58 32,35.31 27.69,35.31 26.67,36.32 23.88,36.32 22.86,35.31 5.33,35.31 4.83,34.8 4.83,32.26 5.33,31.75 9.14,31.75 12.7,28.19 R41.2 | R41.2 C3.2 | R41.2 12.7,27.69
N$47
  Bottom 0.61: U$19.5 10.05,38.47 8.38,40.13 4.83,40.13 4.32,40.64 4.32,50.43 U$2.5
N$48
  Top 0.305: Q1.3 33.05,56.83 C4.1 33.95,56.48 34.54,55.88 34.54,53.85 33.78,53.09 32.51,53.09 31.97,52.55 U$3.10
N$49
  Top 0.305: U$3.11 31.17,52.65 30.73,53.09 28.96,53.09 27.62,54.43 Q1.1 24.99,54.43 C5.1
N$50
  Top 0.61: R17.2 U$4.P$3
N$51
  Top 0.254: R16.1 3.52,18.58 3.05,19.05 3.05,21.34 4.83,21.34 5.33,21.84 6.6,21.84 8.13,23.37 8.13,27.48 U$6.P$1
  Top 0.61: U$18.1 4.83,3.81 3.05,5.59 3.05,15.56 U$4.P$2 4.33,18.44 R16.1
N$52
  Top 0.61: R13.1 6.33,18.44 U$4.P$1
N$53
  Top 0.61: 21.34,7.11 21.34,15.56 U$9.P$2 22.62,18.44 R7.1 | U$18.5 21.34,5.95 21.34,7.11 | R31.1 21.34,7.11
N$54
  Top 0.61: R31.2 U$8.P$3
N$55
  Top 0.61: R6.1 20.05,18.44 U$8.P$1
N$56
  Top 0.61: R20.1 15.48,18.44 U$7.P$1
N$57
  Top 0.61: R8.1 24.62,18.44 U$9.P$1
N$58
  Top 0.61: R10.1 29.21,18.71 29.21,19.05 29.19,19.03 U$10.P$1
N$59
  Top 0.61: R12.1 33.77,18.44 U$11.P$1
N$60
  Top 0.61: R28.1 56.63,18.44 U$17.P$1
N$61
  Top 0.61: R19.1 38.34,18.44 U$12.P$1
N$62
  Top 0.61: R22.1 42.91,18.44 U$13.P$1
N$63
  Top 0.61: R24.1 47.48,18.44 U$15.P$1
N$64
  Top 0.61: R26.1 52.05,18.44 U$16.P$1
N$65
  Top 0.61: U$18.12 51.05,6.88 R38.1 53.34,7.11 53.34,15.56 U$17.P$2 54.63,18.44 R27.1
N$66  (via drill 0.6)
  Top 0.254: U$1.30 32.23,31.27 33.02,30.48 v33.78,30.48 38.14,30.48 | 38.14,30.48 v41.4,30.48 | 38.14,30.48 C14.1 | R55.2 45.47,29.46 v44.45,30.48 | v32.26,28.96 31.75,28.45 24.89,28.45 23.37,26.92 19.39,26.92 R15.2
  Bottom 0.254: v41.4,30.48 v44.45,30.48 | v32.26,28.96 v33.78,30.48
N$67
  Top 0.254: U$1.28 33.23,34.75 34.29,35.81 41.91,35.81 44.2,33.53 C19.2 R40.2
N$68
  Top 0.305: LD1.AR 41.4,47.24 40.39,46.23 R29.1
N$69
  Top 0.61: U$18.11 46.48,5.81 R37.1 48.77,7.11 48.77,15.56 U$16.P$2 50.05,18.44 R25.1
N$70
  Top 0.61: U$18.10 41.91,4.74 R36.1 44.2,7.11 44.2,15.56 U$15.P$2 45.48,18.44 R23.1
N$71
  Top 0.61: U$16.P$3 R38.2
N$72
  Top 0.61: U$17.P$3 R39.2
N$73
  Top 0.61: U$15.P$3 R37.2
N$74
  Top 0.61: 39.62,7.11 39.62,5.95 U$18.9 | 39.62,7.11 R35.1 | 39.62,7.11 39.62,15.56 U$13.P$2 40.91,18.44 R21.1
N$75
  Top 0.61: U$13.P$3 R36.2
N$76
  Top 0.61: 35.05,7.11 35.05,15.56 U$12.P$2 36.34,18.44 R18.1 | U$18.8 35.05,4.88 35.05,7.11 | 35.05,7.11 R34.1
N$77
  Top 0.61: U$12.P$3 R35.2
N$78
  Top 0.61: 30.48,7.11 30.48,15.56 U$11.P$2 31.77,18.44 R11.1 | 30.48,7.11 R33.1 | U$18.7 30.48,7.11
N$79
  Top 0.61: U$18.6 25.91,4.88 25.91,7.11 | 25.91,7.11 25.91,15.56 U$10.P$2 27.19,18.44 R9.1 | 25.91,7.11 R32.1
N$80
  Top 0.61: U$10.P$3 R33.2
N$81
  Top 0.61: U$11.P$3 R34.2
N$82
  Top 0.61: U$9.P$3 R32.2
N$83
  Top 0.254: U$1.21 35.23,24.97 36.83,23.37 44.54,23.37 R24.2
N$84
  Top 0.254: U$1.19 34.23,24.44 36.32,22.35 40.98,22.35 R22.2
N$85
  Top 0.254: R55.1 R40.1 53.11,31.5 U$20.2
N$86
  Top 0.254: R15.1 R41.1 14.48,28.28 14.48,28.7 13.72,29.46 12.19,29.46 8.16,33.5 U$21.2
N$87
  Top 0.254: U$1.7 28.23,24.93 26.67,23.37 23.11,23.37 22.1,22.35 19.3,22.35 18.29,21.34 16.68,21.34 R20.2
N$88
  Top 0.254: U$1.9 29.23,24.4 27.18,22.35 23.62,22.35 22.61,21.34 21.25,21.34 R6.2
N$89
  Top 0.254: R8.2 25.82,21.34 27.69,21.34 30.23,23.88 U$1.11
N$90
  Top 0.254: U$1.13 31.23,23.36 29.34,21.46 R10.2
N$91
  Top 0.254: U$1.15 32.23,21.96 R12.2
N$93
  Top 0.254: U$1.17 33.23,23.92 35.81,21.34 37.43,21.34 R19.2
V+
  Top 0.254: U$1.1 25.23,26.42 17.87,26.42 C13.1 17.61,25.23 16.76,24.38 10.62,24.38 U$6.P$2
VIA
  Top 0.305: U$14.3 18.41,41.91 20.57,44.07 26.54,44.07 27.17,43.44 U$3.25
VIB
  Top 0.305: U$14.4 17.14,41.91 19.94,44.7 25.55,44.7 U$3.24
VIC
  Top 0.305: U$14.5 15.88,41.91 19.3,45.34 24.51,45.34 24.8,45.62 U$3.23
VOD
  Top 0.305: U$3.22 25.67,46.35 24.51,46.35 24.13,45.97 18.67,45.97 14.61,41.91 U$14.6
  Top 0.406: U$14.6 14.73,41.27

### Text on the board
tPlace: MODULE ID | STATUS | GND | ZEVA BMS12 v3.1 (OS Edition) | 12-cell Lithium Battery Management Module | + | -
